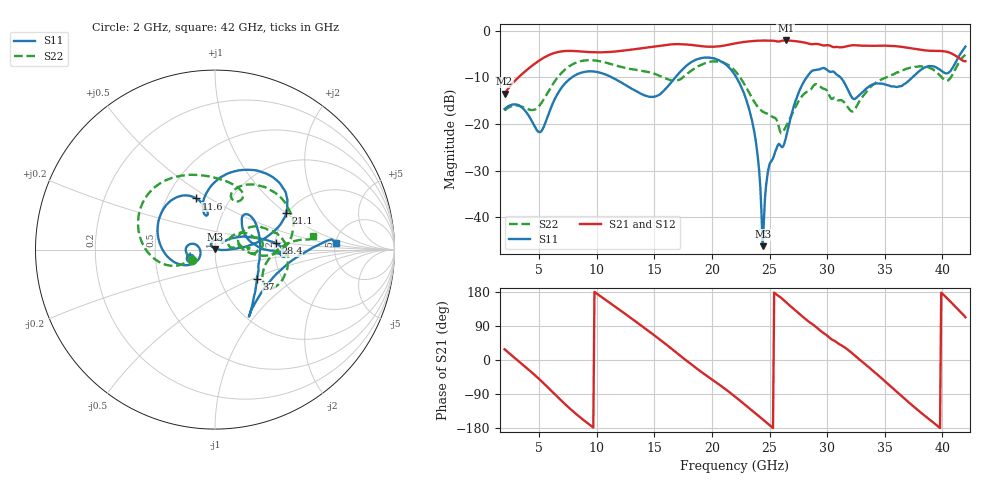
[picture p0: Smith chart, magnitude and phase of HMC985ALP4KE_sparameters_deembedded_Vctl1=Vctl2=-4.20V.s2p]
!s2p File: Measurements: S11, S21, S12, S22
# GHz S dB R 50.0
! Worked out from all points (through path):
!   401 points, 2 GHz to 42 GHz, reference 50 ohm
!   highest |S21| = -2.08 dB at 26.4 GHz (marker M1); lowest = -13.5 dB at 2 GHz (marker M2)
!   lowest |S11| = -46.1 dB at 24.4 GHz (marker M3), VSWR 1.01, Z = 50.3 + j0.415 ohm
!   |S11| at or under -10 dB: start of sweep to 7.832 GHz; 22.12 GHz to 28.22 GHz (6.095 GHz wide, 24.2 % of centre); 31.16 GHz to 37.39 GHz (6.233 GHz wide, 18.2 % of centre)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
!   |S22| runs from -21.9 to -5.2 dB; largest |S21 - S12| = 0.00069
!   S11 on the Smith chart (normalised r, x): 2 GHz: 0.75, -0.07; 11.6 GHz: 0.70, +0.44; 21.1 GHz: 1.98, +1.00; 28.4 GHz: 2.01, +0.16; 37 GHz: 1.50, -0.53; 42 GHz: 5.09, +0.65
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2  -16.78 -162.0  -13.45 28.1  -13.46 28.1  -17.09 -155.9
5  -21.72 -174.2  -6.40 -50.3  -6.40 -50.3  -16.11 -160.6
6.3  -14.91 -151.1  -4.78 -88.5  -4.78 -88.5  -11.02 -162.2
8.7  -8.95 149.9  -4.45 -154.8  -4.45 -154.8  -6.46 150.9
11.6  -10.36 110.1  -4.45 140.6  -4.45 140.6  -7.40 103.0
13.6  -13.19 101.5  -3.85 96.6  -3.85 96.6  -8.45 75.3
15.4  -13.74 106.6  -3.24 55.7  -3.24 55.7  -9.59 62.0
17.9  -7.25 79.6  -2.96 -4.5  -2.96 -4.5  -9.11 72.0
21.1  -7.04 27.0  -3.15 -75.3  -3.16 -75.3  -6.92 15.3
22  -9.49 16.5  -2.72 -96.6  -2.72 -96.6  -8.57 -0.0
23.6  -20.71 1.1  -2.19 -136.4  -2.19 -136.4  -14.92 -3.8
24.4  -46.15 56.9  -2.10 -156.6  -2.10 -156.6  -17.32 8.2
25  -28.58 128.2  -2.12 -171.9  -2.13 -171.9  -17.96 11.9
26.4  -23.12 41.6  -2.08 153.3  -2.08 153.4  -20.61 33.7
28.4  -9.37 6.1  -2.75 101.3  -2.75 101.3  -12.89 17.6
28.7  -8.57 1.1  -2.89 95.1  -2.89 95.1  -12.18 15.8
32.4  -14.62 29.9  -3.10 11.7  -3.10 11.7  -16.84 26.4
33.9  -11.55 48.2  -3.22 -26.5  -3.22 -26.5  -11.75 30.2
35.4  -11.76 17.9  -3.22 -66.5  -3.22 -66.5  -9.73 18.8
37  -10.89 -34.9  -3.64 -109.6  -3.64 -109.5  -8.07 4.1
39.8  -8.36 -56.3  -4.33 -179.6  -4.33 -179.6  -9.58 -34.7
42  -3.40 2.9  -6.52 112.8  -6.52 112.8  -5.15 7.8
